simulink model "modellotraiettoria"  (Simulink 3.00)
settings: Solver=ode45  StartTime=0.0  StopTime=10.0  RelTol=1e-3
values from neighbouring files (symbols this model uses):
  a = u(9)    [acceler.m]    (also in Dati2lin.m = 1; cin_inversa.m = u(4))
  b1 = 1    [Dati2lin.m]
  b2 = 1    [Dati2lin.m]
  Del1 = 0.0022    [Dati2lin.m]
  Del2 = 0.0022    [Dati2lin.m]
  Dm1 = 0.000172    [Dati2lin.m]
  Dm2 = 0.000071    (= 7.1e-05)    [Dati2lin.m]
  g = u(10)    [acceler.m]    (also in Dati2lin.m = 9.806)
  Jm1 = 0.000656    [Dati2lin.m]
  Jm2 = 0.000027    (= 2.7e-05)    [Dati2lin.m]
  Kcp1 = 32    [Dati2lin.m]
  Kcp2 = 32    [Dati2lin.m]
  Kcv1 = 0.24275    [Dati2lin.m]
  Kcv2 = 0.029363    [Dati2lin.m]
  Ke1 = 1.43    [Dati2lin.m]
  Ke2 = 0.79    [Dati2lin.m]
  Kel1 = 36.3    [Dati2lin.m]
  Kel2 = 4.6    [Dati2lin.m]
  Kt1 = 1.75    [Dati2lin.m]
  Kt2 = 0.97    [Dati2lin.m]
  L1 = 0.060    (= 0.06)    [Dati2lin.m]
  L2 = 0.0438    [Dati2lin.m]
  m1 = u(7)    [acceler.m]    (also in Dati2lin.m = 19)
  m2 = u(8)    [acceler.m]    (also in Dati2lin.m = 9)
  n1 = 100    [Dati2lin.m]
  n2 = 100    [Dati2lin.m]
  q01 = atan2(s1,c1)    [traiettoria1.m]    (also in traiettoria2.m; traiettoria3.m; Dati2lin.m = 0)
  q02 = atan2(s2,c2)    [traiettoria1.m]    (also in traiettoria2.m; traiettoria3.m; Dati2lin.m = 0)
  qm01 = n1*q01 + taulm01/Kel1    [traiettoria1.m]    (also in traiettoria2.m; traiettoria3.m; Dati2lin.m)
  qm02 = n2*q02 + taulm02/Kel2    [traiettoria1.m]    (also in traiettoria2.m; traiettoria3.m; Dati2lin.m)
  R1 = 3.3    [Dati2lin.m]
  R2 = 20.4    [Dati2lin.m]
  Tiv1 = 25    [Dati2lin.m]
  Tiv2 = 5.2632    [Dati2lin.m]
  u01 = taulm01/Kt1    [traiettoria1.m]    (also in traiettoria2.m; traiettoria3.m; Dati2lin.m)
  u02 = taulm02/Kt2    [traiettoria1.m]    (also in traiettoria2.m; traiettoria3.m; Dati2lin.m)

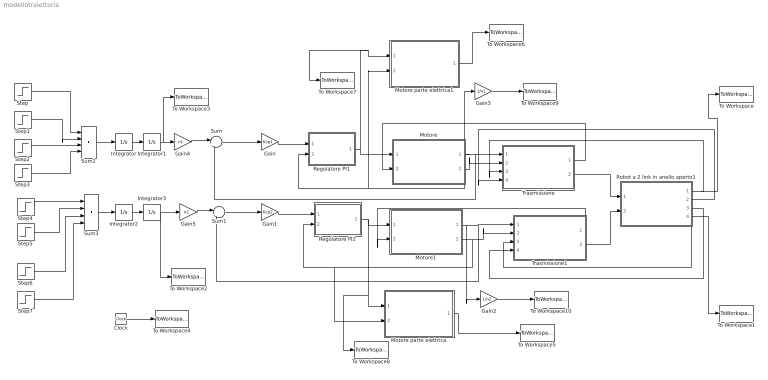
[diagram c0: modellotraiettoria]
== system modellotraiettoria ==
  Clock : Clock
  Gain : Gain  Gain=Kcp1  SaturateOnIntegerOverflow=on
  Gain1 : Gain  Gain=Kcp2  SaturateOnIntegerOverflow=on
  Gain2 : Gain  Gain=1/n2  SaturateOnIntegerOverflow=on
  Gain3 : Gain  Gain=1/n1  SaturateOnIntegerOverflow=on
  Gain4 : Gain  Gain=n1  SaturateOnIntegerOverflow=on
  Gain5 : Gain  Gain=n2  SaturateOnIntegerOverflow=on
  Integrator{,1..3} (4 alike) : Integrator  ExternalReset=none  InitialConditionSource=internal  InitialCondition=0  LimitOutput=off  UpperSaturationLimit=inf  LowerSaturationLimit=-inf  ShowSaturationPort=off  ShowStatePort=off  AbsoluteTolerance=auto
  Motore : Subsystem  mask(Motore (solo meccanica)){Kt=Kt1, Jm=Jm1, Dm=Dm1, Qm0=qm01}
      mask prompts: Kt "Costante di coppia (Kt)"; Jm "Momento d'inerzia (Jm)"; Dm "Coefficiente di attrito viscoso (Dm)"; Qm0 "Posizione iniziale (Qm0)"
      mask help: Motore controllato in tensione - Modello che tiene conto degli effetti dell'attrito (solo quello viscoso)
  Motore parte elettrica : Subsystem  mask(Motore - parte elettrica){Ke=Ke2, R=R2, L=L2}
      mask prompts: Ke "Costante di forza controelettromotrice (Ke)"; R "Resistenza (R)"; L "Induttanza (L)"
      mask help: Motore - elettrica per calcolare la tensione da imporre ai morsetti, per ottenere corrente necessaria ad attuare il moto desiderato
  Motore parte elettrica1 : Subsystem  mask(Motore - parte elettrica){Ke=Ke1, R=R1, L=L1}
      mask prompts: Ke "Costante di forza controelettromotrice (Ke)"; R "Resistenza (R)"; L "Induttanza (L)"
      mask help: Motore - elettrica per calcolare la tensione da imporre ai morsetti, per ottenere corrente necessaria ad attuare il moto desiderato
  Motore1 : Subsystem  mask(Motore (solo meccanica)){Kt=Kt2, Jm=Jm2, Dm=Dm2, Qm0=qm02}
      mask prompts: Kt "Costante di coppia (Kt)"; Jm "Momento d'inerzia (Jm)"; Dm "Coefficiente di attrito viscoso (Dm)"; Qm0 "Posizione iniziale (Qm0)"
      mask help: Motore controllato in tensione - Modello che tiene conto degli effetti dell'attrito (solo quello viscoso)
  Regolatore PI1 : Subsystem  mask(Controllore PID ISA){Kc=Kcv1, Ti=Tiv1, b=b1, p6=[-inf,inf], u0=u01}
      mask prompts: Kc "Guadagno (Kc)"; Ti "Tempo integrale (Ti)"; b "Peso sul setpoint (b)"; p6 "Saturazione antiwindup ([umin, umax])"; u0 "Variabile di controllo iniziale (u0)"
      mask init:
      | ulow = p6(1);
      | uhigh = p6(2);
  Regolatore PI2 : Subsystem  mask(Controllore PID ISA){Kc=Kcv2, Ti=Tiv2, b=b2, p6=[-inf,inf], u0=u02}
      mask prompts: Kc "Guadagno (Kc)"; Ti "Tempo integrale (Ti)"; b "Peso sul setpoint (b)"; p6 "Saturazione antiwindup ([umin, umax])"; u0 "Variabile di controllo iniziale (u0)"
      mask init:
      | ulow = p6(1);
      | uhigh = p6(2);
  Robot a 2 link in anello aperto1 : Subsystem  mask(Modello del robot planare a 2 link){m1=m1, m2=m2, a=a, q01=q01, q02=q02, g=g}
      mask prompts: m1 "Massa del link 1 (m1)"; m2 "Massa del link 2 (m2)"; a "Lunghezza del link (a)"; q01 "Posizione iniziale link 1 (q01)"; q02 "Posizione iniziale link 2 (q02)"; g "Accelerazione di gravità (g)"
  Step : Step  Time=0  Before=15  After=15  SampleTime=0
  Step1 : Step  Time=0.2  Before=0  After=-15  SampleTime=0
  Step2 : Step  Time=0.67  Before=0  After=-15  SampleTime=0
  Step3 : Step  Time=0.87  Before=0  After=15  SampleTime=0
  Step4 : Step  Time=0  Before=0  After=0  SampleTime=0
  Step5 : Step  Time=0.2  Before=0  After=0  SampleTime=0
  Step6 : Step  Time=0.67  Before=0  After=0  SampleTime=0
  Step7 : Step  Time=0.87  Before=0  After=0  SampleTime=0
  Sum : Sum  Inputs=|+-  SaturateOnIntegerOverflow=on
  Sum1 : Sum  Inputs=|+-  SaturateOnIntegerOverflow=on
  Sum2 : Sum  Inputs=|++++  SaturateOnIntegerOverflow=on
  Sum3 : Sum  Inputs=|++++  SaturateOnIntegerOverflow=on
  To Workspace : ToWorkspace  VariableName=qout1  SampleTime=-1  SaveFormat=Matrix
  To Workspace1 : ToWorkspace  VariableName=qout2  SampleTime=-1  SaveFormat=Matrix
  To Workspace10 : ToWorkspace  VariableName=qmout2  SampleTime=-1  SaveFormat=Matrix
  To Workspace2 : ToWorkspace  VariableName=setlink2  SampleTime=-1  SaveFormat=Matrix
  To Workspace3 : ToWorkspace  VariableName=setlink1  SampleTime=-1  SaveFormat=Matrix
  To Workspace4 : ToWorkspace  VariableName=x  SampleTime=-1  SaveFormat=Matrix
  To Workspace5 : ToWorkspace  VariableName=Vm2  SampleTime=-1  SaveFormat=Matrix
  To Workspace6 : ToWorkspace  VariableName=Vm1  SampleTime=-1  SaveFormat=Matrix
  To Workspace7 : ToWorkspace  VariableName=Im1  SampleTime=-1  SaveFormat=Matrix
  To Workspace8 : ToWorkspace  VariableName=Im2  SampleTime=-1  SaveFormat=Matrix
  To Workspace9 : ToWorkspace  VariableName=qmout1  SampleTime=-1  SaveFormat=Matrix
  Trasmissione : Subsystem  mask(Riduttore){n=n1, Kel=Kel1, Del=Del1}
      mask prompts: n "Rapporto di trasmissione (n)"; Kel "Coefficiente di elasticità (Kel)"; Del "Coefficiente di smorzamento (Del)"
      mask help: Riduttore - Modello che tiene conto dei soli effetti elastici (senza considerare le inerzie, accorpate nel modello del motore) e di un termine di smorzamento
  Trasmissione1 : Subsystem  mask(Riduttore){n=n2, Kel=Kel2, Del=Del2}
      mask prompts: n "Rapporto di trasmissione (n)"; Kel "Coefficiente di elasticità (Kel)"; Del "Coefficiente di smorzamento (Del)"
      mask help: Riduttore - Modello che tiene conto dei soli effetti elastici (senza considerare le inerzie, accorpate nel modello del motore) e di un termine di smorzamento
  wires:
  Sum/1 -> Gain/1
  Sum1/1 -> Gain1/1
  Gain/1 -> Regolatore PI1/1(ysp)
  Gain1/1 -> Regolatore PI2/1(ysp)
  Trasmissione/2("tau_ll ") -> Robot a 2 link in anello aperto1/1(taull1)
  Trasmissione1/2("tau_ll ") -> Robot a 2 link in anello aperto1/2(taull2)
  Trasmissione1/1("tau_lm ") -> Motore1/2(tau_lm)
  Robot a 2 link in anello aperto1/3(dq2) -> Trasmissione1/4("dq ")
  Robot a 2 link in anello aperto1/2(dq1) -> Trasmissione/4("dq ")
  Trasmissione/1("tau_lm ") -> Motore/2(tau_lm)
  Motore1/2(dqm) -> Trasmissione1/2(dqm), Regolatore PI2/2(y), Motore parte elettrica/2(dqm)
  Motore/2(dqm) -> Trasmissione/2(dqm), Regolatore PI1/2(y), Motore parte elettrica1/2(dqm)
  Robot a 2 link in anello aperto1/4(q2) -> Trasmissione1/3("q "), To Workspace1/1
  Robot a 2 link in anello aperto1/1(q1) -> Trasmissione/3("q "), To Workspace/1
  Motore/1(qm) -> Trasmissione/1(qm), Sum/2, Gain3/1
  Motore1/1(qm) -> Trasmissione1/1(qm), Sum1/2, Gain2/1
  Integrator2/1 -> Integrator3/1
  Integrator/1 -> Integrator1/1
  Sum2/1 -> Integrator/1
  Sum3/1 -> Integrator2/1
  Step/1 -> Sum2/1
  Step2/1 -> Sum2/3
  Step3/1 -> Sum2/4
  Step4/1 -> Sum3/1
  Step5/1 -> Sum3/2
  Step6/1 -> Sum3/3
  Step7/1 -> Sum3/4
  Step1/1 -> Sum2/2
  Gain4/1 -> Sum/1
  Gain5/1 -> Sum1/1
  Integrator3/1 -> To Workspace2/1, Gain5/1
  Clock/1 -> To Workspace4/1
  Regolatore PI2/1(u) -> Motore1/1(I), Motore parte elettrica/1(I), To Workspace8/1
  Regolatore PI1/1(u) -> Motore/1(I), Motore parte elettrica1/1(I), To Workspace7/1
  Motore parte elettrica1/1(V) -> To Workspace6/1
  Motore parte elettrica/1(V) -> To Workspace5/1
  Gain3/1 -> To Workspace9/1
  Gain2/1 -> To Workspace10/1
  Integrator1/1 -> Gain4/1, To Workspace3/1

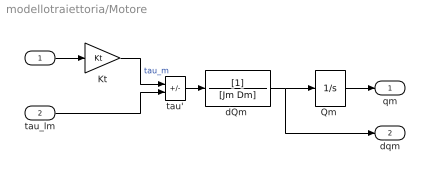
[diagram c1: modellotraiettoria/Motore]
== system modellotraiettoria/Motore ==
  I : Inport  Port=1  PortWidth=-1  SampleTime=-1  DataType=auto
  tau_lm : Inport  Port=2  PortWidth=-1  SampleTime=-1  DataType=auto
  Kt : Gain  Gain=Kt  SaturateOnIntegerOverflow=on
  "Qm " : Integrator  ExternalReset=none  InitialConditionSource=internal  InitialCondition=Qm0  LimitOutput=off  UpperSaturationLimit=inf  LowerSaturationLimit=-inf  ShowSaturationPort=off  ShowStatePort=off  AbsoluteTolerance=auto
  "dQm " : TransferFcn  Numerator=[1]  Denominator=[Jm Dm]
  tau' : Sum  Inputs=+-  SaturateOnIntegerOverflow=on
  qm : Outport  Port=1
  dqm : Outport  Port=2
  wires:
  "Qm "/1 -> qm/1
  "dQm "/1 -> dqm/1, "Qm "/1
  tau'/1 -> "dQm "/1
  Kt/1 -> tau'/1  "tau_m"
  I/1 -> Kt/1
  tau_lm/1 -> tau'/2

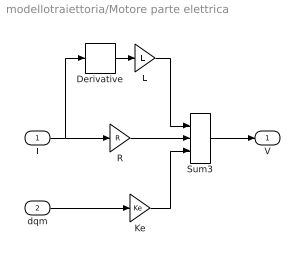
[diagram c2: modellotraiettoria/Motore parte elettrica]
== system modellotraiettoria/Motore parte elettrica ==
  I : Inport  Port=1  PortWidth=-1  SampleTime=-1  DataType=auto
  dqm : Inport  Port=2  PortWidth=-1  SampleTime=-1  DataType=auto
  Derivative : Derivative
  Ke : Gain  Gain=Ke  SaturateOnIntegerOverflow=on
  L : Gain  Gain=L  SaturateOnIntegerOverflow=on
  R : Gain  Gain=R  SaturateOnIntegerOverflow=on
  Sum3 : Sum  Inputs=+++  SaturateOnIntegerOverflow=on
  V : Outport  Port=1
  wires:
  Sum3/1 -> V/1
  Ke/1 -> Sum3/3
  Derivative/1 -> L/1
  L/1 -> Sum3/1
  I/1 -> Derivative/1, R/1
  R/1 -> Sum3/2
  dqm/1 -> Ke/1

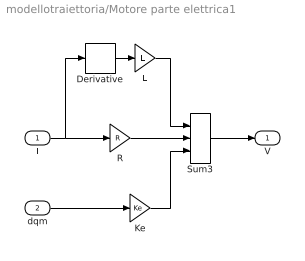
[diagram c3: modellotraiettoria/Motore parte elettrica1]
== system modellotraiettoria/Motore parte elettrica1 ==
  I : Inport  Port=1  PortWidth=-1  SampleTime=-1  DataType=auto
  dqm : Inport  Port=2  PortWidth=-1  SampleTime=-1  DataType=auto
  Derivative : Derivative
  Ke : Gain  Gain=Ke  SaturateOnIntegerOverflow=on
  L : Gain  Gain=L  SaturateOnIntegerOverflow=on
  R : Gain  Gain=R  SaturateOnIntegerOverflow=on
  Sum3 : Sum  Inputs=+++  SaturateOnIntegerOverflow=on
  V : Outport  Port=1
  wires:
  Sum3/1 -> V/1
  Ke/1 -> Sum3/3
  Derivative/1 -> L/1
  L/1 -> Sum3/1
  I/1 -> Derivative/1, R/1
  R/1 -> Sum3/2
  dqm/1 -> Ke/1

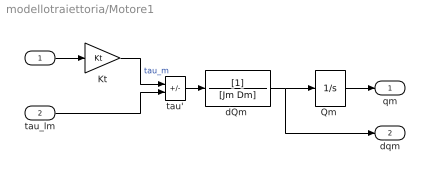
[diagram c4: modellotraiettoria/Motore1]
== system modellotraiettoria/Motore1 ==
  I : Inport  Port=1  PortWidth=-1  SampleTime=-1  DataType=auto
  tau_lm : Inport  Port=2  PortWidth=-1  SampleTime=-1  DataType=auto
  Kt : Gain  Gain=Kt  SaturateOnIntegerOverflow=on
  "Qm " : Integrator  ExternalReset=none  InitialConditionSource=internal  InitialCondition=Qm0  LimitOutput=off  UpperSaturationLimit=inf  LowerSaturationLimit=-inf  ShowSaturationPort=off  ShowStatePort=off  AbsoluteTolerance=auto
  "dQm " : TransferFcn  Numerator=[1]  Denominator=[Jm Dm]
  tau' : Sum  Inputs=+-  SaturateOnIntegerOverflow=on
  qm : Outport  Port=1
  dqm : Outport  Port=2
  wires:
  "Qm "/1 -> qm/1
  "dQm "/1 -> dqm/1, "Qm "/1
  tau'/1 -> "dQm "/1
  Kt/1 -> tau'/1  "tau_m"
  I/1 -> Kt/1
  tau_lm/1 -> tau'/2

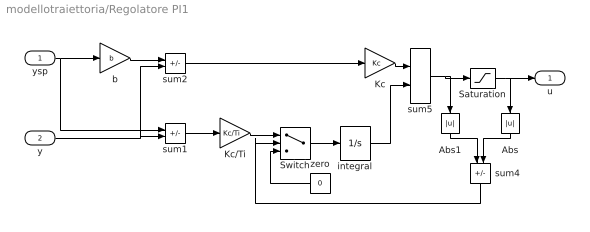
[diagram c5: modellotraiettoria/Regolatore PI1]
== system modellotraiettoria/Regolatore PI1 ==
  ysp : Inport  Port=1  PortWidth=-1  SampleTime=-1  DataType=auto
  y : Inport  Port=2  PortWidth=-1  SampleTime=-1  DataType=auto
  Abs : Abs  Orientation=down
  Abs1 : Abs  Orientation=down
  Kc : Gain  Gain=Kc  SaturateOnIntegerOverflow=on
  Kc/Ti : Gain  Gain=Kc/Ti  SaturateOnIntegerOverflow=on
  Saturation : Saturate  UpperLimit=uhigh  LowerLimit=ulow
  Switch : Switch  Threshold=0
  b : Gain  Gain=b  SaturateOnIntegerOverflow=on
  integral : Integrator  ExternalReset=none  InitialConditionSource=internal  InitialCondition=u0  LimitOutput=off  UpperSaturationLimit=inf  LowerSaturationLimit=-inf  ShowSaturationPort=off  ShowStatePort=off  AbsoluteTolerance=auto
  sum1 : Sum  Inputs=+-  SaturateOnIntegerOverflow=on
  sum2 : Sum  Inputs=+-  SaturateOnIntegerOverflow=on
  sum4 : Sum  Orientation=down  Inputs=-+  SaturateOnIntegerOverflow=on
  sum5 : Sum  Inputs=++  SaturateOnIntegerOverflow=on
  zero : Constant  Orientation=left  Value=0
  u : Outport  Port=1
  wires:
  integral/1 -> sum5/2
  sum1/1 -> Kc/Ti/1
  Abs/1 -> sum4/2
  Abs1/1 -> sum4/1
  sum5/1 -> Saturation/1, Abs1/1
  Saturation/1 -> Abs/1, u/1
  Switch/1 -> integral/1
  zero/1 -> Switch/3
  sum4/1 -> Switch/2
  Kc/Ti/1 -> Switch/1
  Kc/1 -> sum5/1
  sum2/1 -> Kc/1
  y/1 -> sum1/2, sum2/2
  b/1 -> sum2/1
  ysp/1 -> sum1/1, b/1

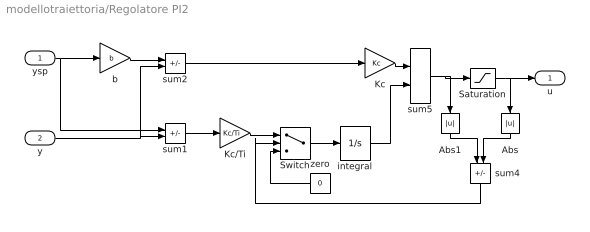
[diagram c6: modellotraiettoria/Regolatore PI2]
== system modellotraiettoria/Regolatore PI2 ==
  ysp : Inport  Port=1  PortWidth=-1  SampleTime=-1  DataType=auto
  y : Inport  Port=2  PortWidth=-1  SampleTime=-1  DataType=auto
  Abs : Abs  Orientation=down
  Abs1 : Abs  Orientation=down
  Kc : Gain  Gain=Kc  SaturateOnIntegerOverflow=on
  Kc/Ti : Gain  Gain=Kc/Ti  SaturateOnIntegerOverflow=on
  Saturation : Saturate  UpperLimit=uhigh  LowerLimit=ulow
  Switch : Switch  Threshold=0
  b : Gain  Gain=b  SaturateOnIntegerOverflow=on
  integral : Integrator  ExternalReset=none  InitialConditionSource=internal  InitialCondition=u0  LimitOutput=off  UpperSaturationLimit=inf  LowerSaturationLimit=-inf  ShowSaturationPort=off  ShowStatePort=off  AbsoluteTolerance=auto
  sum1 : Sum  Inputs=+-  SaturateOnIntegerOverflow=on
  sum2 : Sum  Inputs=+-  SaturateOnIntegerOverflow=on
  sum4 : Sum  Orientation=down  Inputs=-+  SaturateOnIntegerOverflow=on
  sum5 : Sum  Inputs=++  SaturateOnIntegerOverflow=on
  zero : Constant  Orientation=left  Value=0
  u : Outport  Port=1
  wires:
  integral/1 -> sum5/2
  sum1/1 -> Kc/Ti/1
  Abs/1 -> sum4/2
  Abs1/1 -> sum4/1
  sum5/1 -> Saturation/1, Abs1/1
  Saturation/1 -> Abs/1, u/1
  Switch/1 -> integral/1
  zero/1 -> Switch/3
  sum4/1 -> Switch/2
  Kc/Ti/1 -> Switch/1
  Kc/1 -> sum5/1
  sum2/1 -> Kc/1
  y/1 -> sum1/2, sum2/2
  b/1 -> sum2/1
  ysp/1 -> sum1/1, b/1

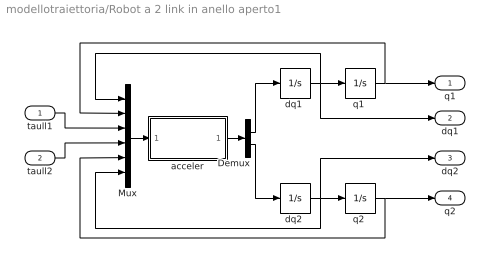
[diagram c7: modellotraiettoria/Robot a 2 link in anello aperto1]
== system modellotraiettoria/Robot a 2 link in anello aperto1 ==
  taull1 : Inport  Port=1  PortWidth=-1  SampleTime=-1  DataType=auto
  taull2 : Inport  Port=2  PortWidth=-1  SampleTime=-1  DataType=auto
  Demux : Demux  Outputs=2
  Mux : Mux  Inputs=6
  acceler : Subsystem
  "dq1 " : Integrator  ExternalReset=none  InitialConditionSource=internal  InitialCondition=0  LimitOutput=off  UpperSaturationLimit=inf  LowerSaturationLimit=-inf  ShowSaturationPort=off  ShowStatePort=off  AbsoluteTolerance=auto
  "dq2 " : Integrator  ExternalReset=none  InitialConditionSource=internal  InitialCondition=0  LimitOutput=off  UpperSaturationLimit=inf  LowerSaturationLimit=-inf  ShowSaturationPort=off  ShowStatePort=off  AbsoluteTolerance=auto
  "q1 " : Integrator  ExternalReset=none  InitialConditionSource=internal  InitialCondition=q01  LimitOutput=off  UpperSaturationLimit=inf  LowerSaturationLimit=-inf  ShowSaturationPort=off  ShowStatePort=off  AbsoluteTolerance=auto
  "q2 " : Integrator  ExternalReset=none  InitialConditionSource=internal  InitialCondition=q02  LimitOutput=off  UpperSaturationLimit=inf  LowerSaturationLimit=-inf  ShowSaturationPort=off  ShowStatePort=off  AbsoluteTolerance=auto
  q1 : Outport  Port=1
  dq1 : Outport  Port=2
  dq2 : Outport  Port=3
  q2 : Outport  Port=4
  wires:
  taull2/1 -> Mux/4
  taull1/1 -> Mux/3
  Mux/1 -> acceler/1(u)
  Demux/2 -> "dq2 "/1
  Demux/1 -> "dq1 "/1
  acceler/1(y) -> Demux/1
  "q2 "/1 -> Mux/5, q2/1
  "q1 "/1 -> Mux/2, q1/1
  "dq2 "/1 -> Mux/6, dq2/1, "q2 "/1
  "dq1 "/1 -> Mux/1, dq1/1, "q1 "/1

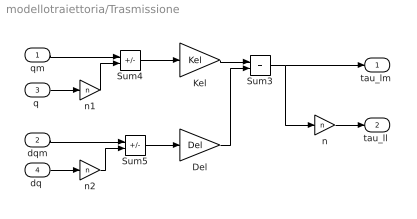
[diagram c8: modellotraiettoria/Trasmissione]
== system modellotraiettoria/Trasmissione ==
  qm : Inport  Port=1  PortWidth=-1  SampleTime=-1  DataType=auto
  dqm : Inport  Port=2  PortWidth=-1  SampleTime=-1  DataType=auto
  "q " : Inport  Port=3  PortWidth=-1  SampleTime=-1  DataType=auto
  "dq " : Inport  Port=4  PortWidth=-1  SampleTime=-1  DataType=auto
  Del : Gain  Gain=Del  SaturateOnIntegerOverflow=on
  Kel : Gain  Gain=Kel  SaturateOnIntegerOverflow=on
  Sum3 : Sum  Inputs=++  SaturateOnIntegerOverflow=on
  Sum4 : Sum  Inputs=+-  SaturateOnIntegerOverflow=on
  Sum5 : Sum  Inputs=+-  SaturateOnIntegerOverflow=on
  n : Gain  Gain=n  SaturateOnIntegerOverflow=on
  n1 : Gain  Gain=n  SaturateOnIntegerOverflow=on
  n2 : Gain  Gain=n  SaturateOnIntegerOverflow=on
  "tau_lm " : Outport  Port=1
  "tau_ll " : Outport  Port=2
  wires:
  Kel/1 -> Sum3/1
  Sum4/1 -> Kel/1
  n1/1 -> Sum4/2
  qm/1 -> Sum4/1
  Sum3/1 -> "tau_lm "/1, n/1
  Del/1 -> Sum3/2
  Sum5/1 -> Del/1
  n/1 -> "tau_ll "/1
  "q "/1 -> n1/1
  n2/1 -> Sum5/2
  dqm/1 -> Sum5/1
  "dq "/1 -> n2/1

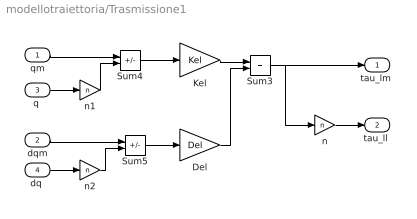
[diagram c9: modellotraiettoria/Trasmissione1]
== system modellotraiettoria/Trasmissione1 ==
  qm : Inport  Port=1  PortWidth=-1  SampleTime=-1  DataType=auto
  dqm : Inport  Port=2  PortWidth=-1  SampleTime=-1  DataType=auto
  "q " : Inport  Port=3  PortWidth=-1  SampleTime=-1  DataType=auto
  "dq " : Inport  Port=4  PortWidth=-1  SampleTime=-1  DataType=auto
  Del : Gain  Gain=Del  SaturateOnIntegerOverflow=on
  Kel : Gain  Gain=Kel  SaturateOnIntegerOverflow=on
  Sum3 : Sum  Inputs=++  SaturateOnIntegerOverflow=on
  Sum4 : Sum  Inputs=+-  SaturateOnIntegerOverflow=on
  Sum5 : Sum  Inputs=+-  SaturateOnIntegerOverflow=on
  n : Gain  Gain=n  SaturateOnIntegerOverflow=on
  n1 : Gain  Gain=n  SaturateOnIntegerOverflow=on
  n2 : Gain  Gain=n  SaturateOnIntegerOverflow=on
  "tau_lm " : Outport  Port=1
  "tau_ll " : Outport  Port=2
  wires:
  Kel/1 -> Sum3/1
  Sum4/1 -> Kel/1
  n1/1 -> Sum4/2
  qm/1 -> Sum4/1
  Sum3/1 -> "tau_lm "/1, n/1
  Del/1 -> Sum3/2
  Sum5/1 -> Del/1
  n/1 -> "tau_ll "/1
  "q "/1 -> n1/1
  n2/1 -> Sum5/2
  dqm/1 -> Sum5/1
  "dq "/1 -> n2/1

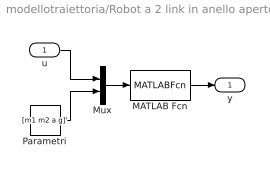
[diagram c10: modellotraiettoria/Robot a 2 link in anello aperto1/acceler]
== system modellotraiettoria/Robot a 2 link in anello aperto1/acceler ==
  u : Inport  Port=1  PortWidth=-1  SampleTime=-1  DataType=auto
  MATLAB Fcn : MATLABFcn  MATLABFcn=acceler  OutputWidth=-1  OutputSignalType=auto
  Mux : Mux  Inputs=2
  Parametri : Constant  Value=[m1 m2 a g]'
  y : Outport  Port=1
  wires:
  MATLAB Fcn/1 -> y/1
  Mux/1 -> MATLAB Fcn/1
  u/1 -> Mux/1
  Parametri/1 -> Mux/2
